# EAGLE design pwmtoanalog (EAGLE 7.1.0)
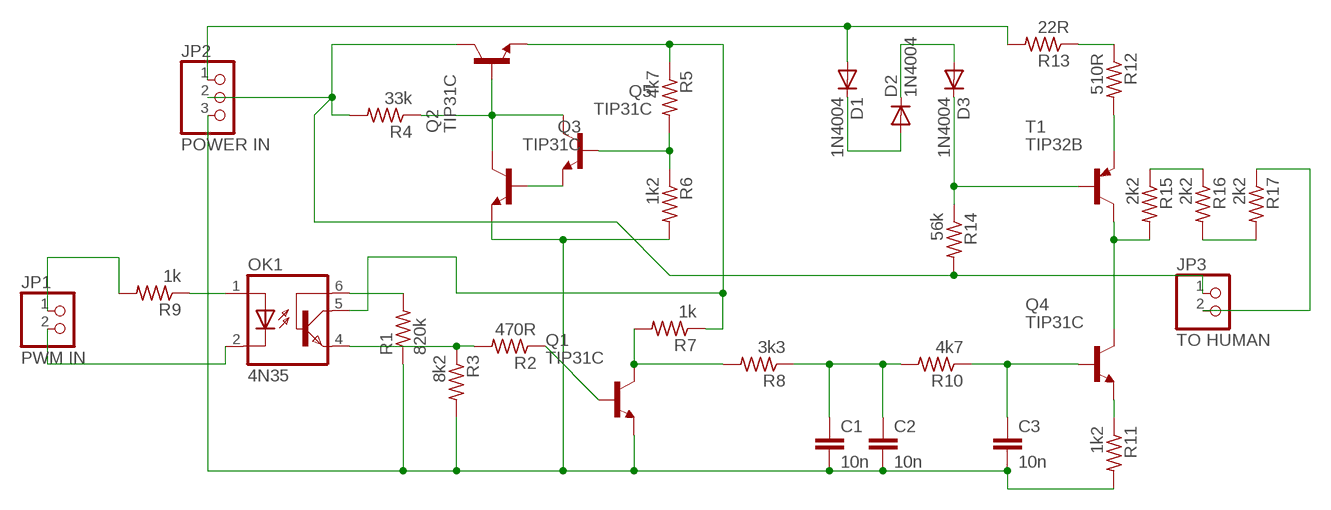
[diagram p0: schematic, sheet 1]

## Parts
C1  10n  C-EU025-030X050  [C025-030X050]
C2  10n  C-EU025-030X050  [C025-030X050]
C3  10n  C-EU025-030X050  [C025-030X050]
D1  1N4004  [DO41-10]
D2  1N4004  [DO41-10]
D3  1N4004  [DO41-10]
JP1  PWM IN  PINHD-1X2  [1X02]
JP2  POWER IN  PINHD-1X3  [1X03]
JP3  TO HUMAN  PINHD-1X2  [1X02]
OK1  4N35  [DIL06]
Q1  TIP31C  [TO220]
Q2  TIP31C  [TO220]
Q3  TIP31C  [TO220]
Q4  TIP31C  [TO220]
Q5  TIP31C  [TO220]
R1  820k  R-US_0207/10  [0207/10]
R2  470R  R-US_0207/10  [0207/10]
R3  8k2  R-US_0207/10  [0207/10]
R4  33k  R-US_0207/10  [0207/10]
R5  4k7  R-US_0207/10  [0207/10]
R6  1k2  R-US_0207/10  [0207/10]
R7  1k  R-US_0207/10  [0207/10]
R8  3k3  R-US_0207/10  [0207/10]
R9  1k  R-US_0207/10  [0207/10]
R10  4k7  R-US_0207/10  [0207/10]
R11  1k2  R-US_0207/10  [0207/10]
R12  510R  R-US_0207/10  [0207/10]
R13  22R  R-US_0207/10  [0207/10]
R14  56k  R-US_0207/10  [0207/10]
R15  2k2  R-US_0207/10  [0207/10]
R16  2k2  R-US_0207/10  [0207/10]
R17  2k2  R-US_0207/10  [0207/10]
T1  TIP32B  [TO220]

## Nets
N$1: OK1.6(BAS) R1.2
N$2: C1.2 C2.2 C3.2 JP2.3 Q1.3(E) Q3.3(E) R1.1 R3.2 R6.2 R11.2
N$3: Q1.1(B) R2.1
N$4: OK1.4(EMI) R2.2 R3.1
N$5: Q2.1(B) Q3.2(C) Q5.2(C) R4.1
N$6: Q3.1(B) Q5.3(E)
N$7: Q5.1(B) R5.2 R6.1
N$8: Q4.3(E) R11.1
N$9: OK1.5(COL) Q2.3(E) R5.1 R7.1
N$10: JP2.2 JP3.1 Q2.2(C) R4.2 R14.2
N$11: Q1.2(C) R7.2 R8.2
N$12: JP1.1 R9.2
N$13: OK1.1(A) R9.1
N$14: JP1.2 OK1.2(C)
N$15: D1.A JP2.1 R13.2
N$16: C3.1 Q4.1(B) R10.1
N$17: C1.1 C2.1 R8.1 R10.2
N$18: R12.1 R13.1
N$19: R12.2 T1.3(E)
N$20: Q4.2(C) R15.2 T1.2(C)
N$21: D3.C R14.1 T1.1(B)
N$22: D1.C D2.A
N$23: D2.C D3.A
N$24: R15.1 R16.1
N$25: R16.2 R17.2
N$26: JP3.2 R17.1

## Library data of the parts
C1-C3 = rcl:C-EU: CAPACITOR, European symbol
D1-D3 = diode:1N4004: DIODE
JP1 JP3 = pinhead:PINHD-1X2: PIN HEADER
JP2 = pinhead:PINHD-1X3: PIN HEADER
OK1 = optocoupler:4N35: MOTOROLA OPTO COUPLER; MF: FAIRCHILD SEMICONDUCTOR; MPN: 4N35; OC_FARNELL: 1328375; OC_NEWARK: 72K9946
Q1-Q5 = transistor-npn:TIP31C*: NPN Transistor
R1-R17 = rcl:R-US_: RESISTOR, American symbol
T1 = transistor:TIP32: PNP Transistor Medium Power Linear Switching Applications Source: http://onsemi.com

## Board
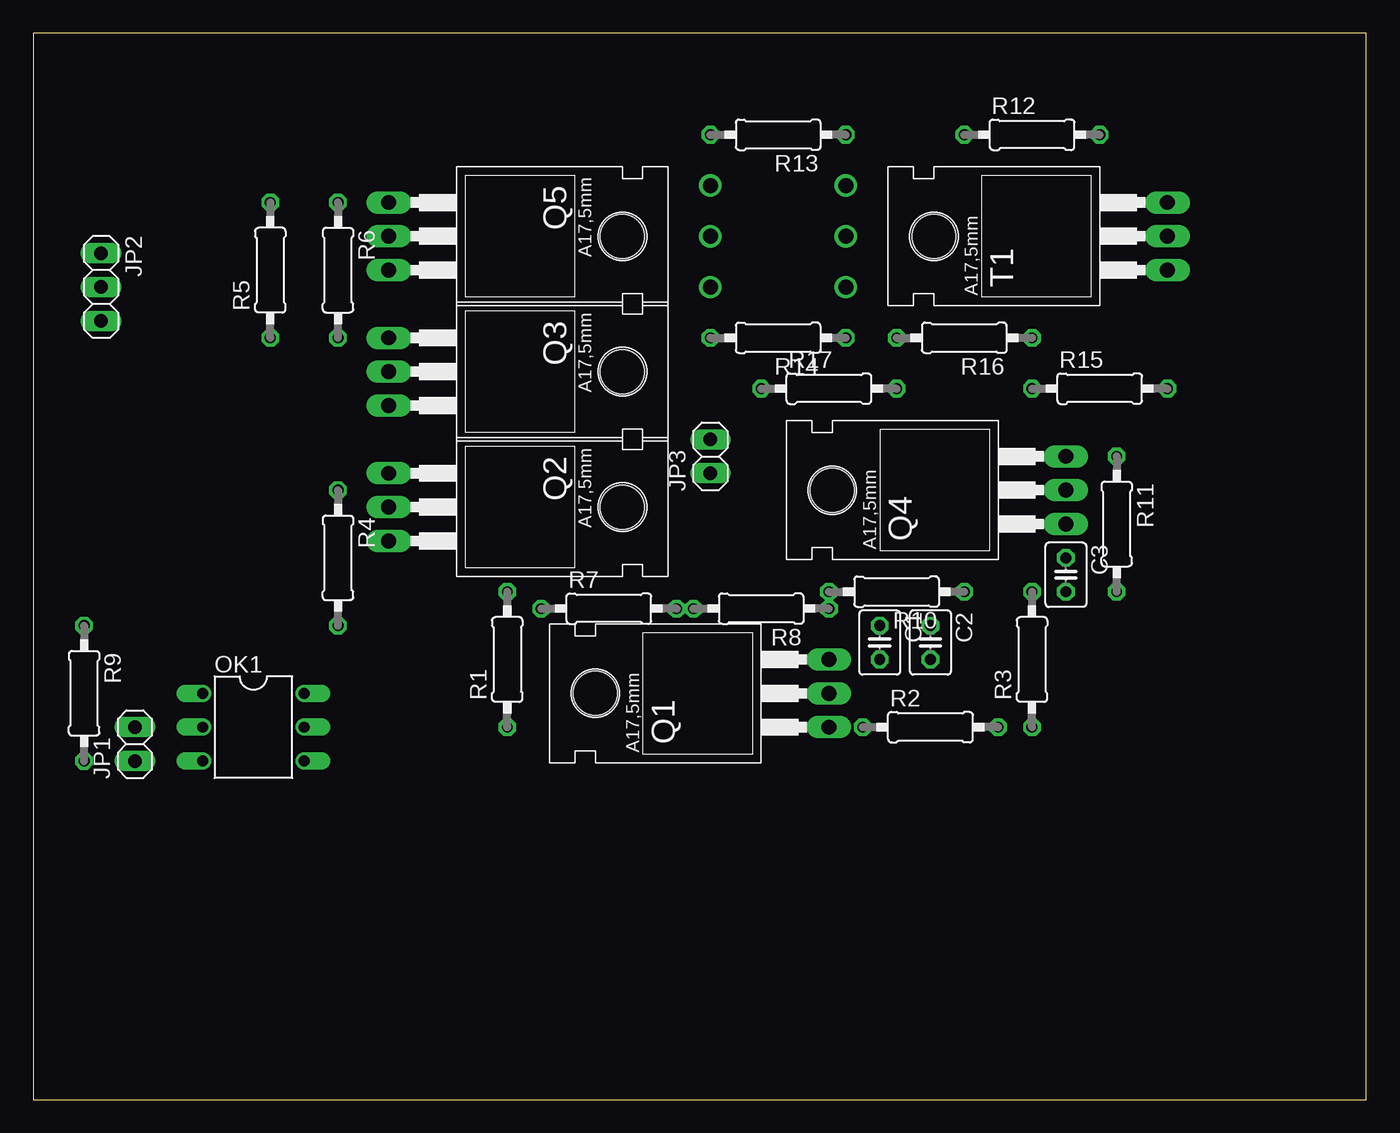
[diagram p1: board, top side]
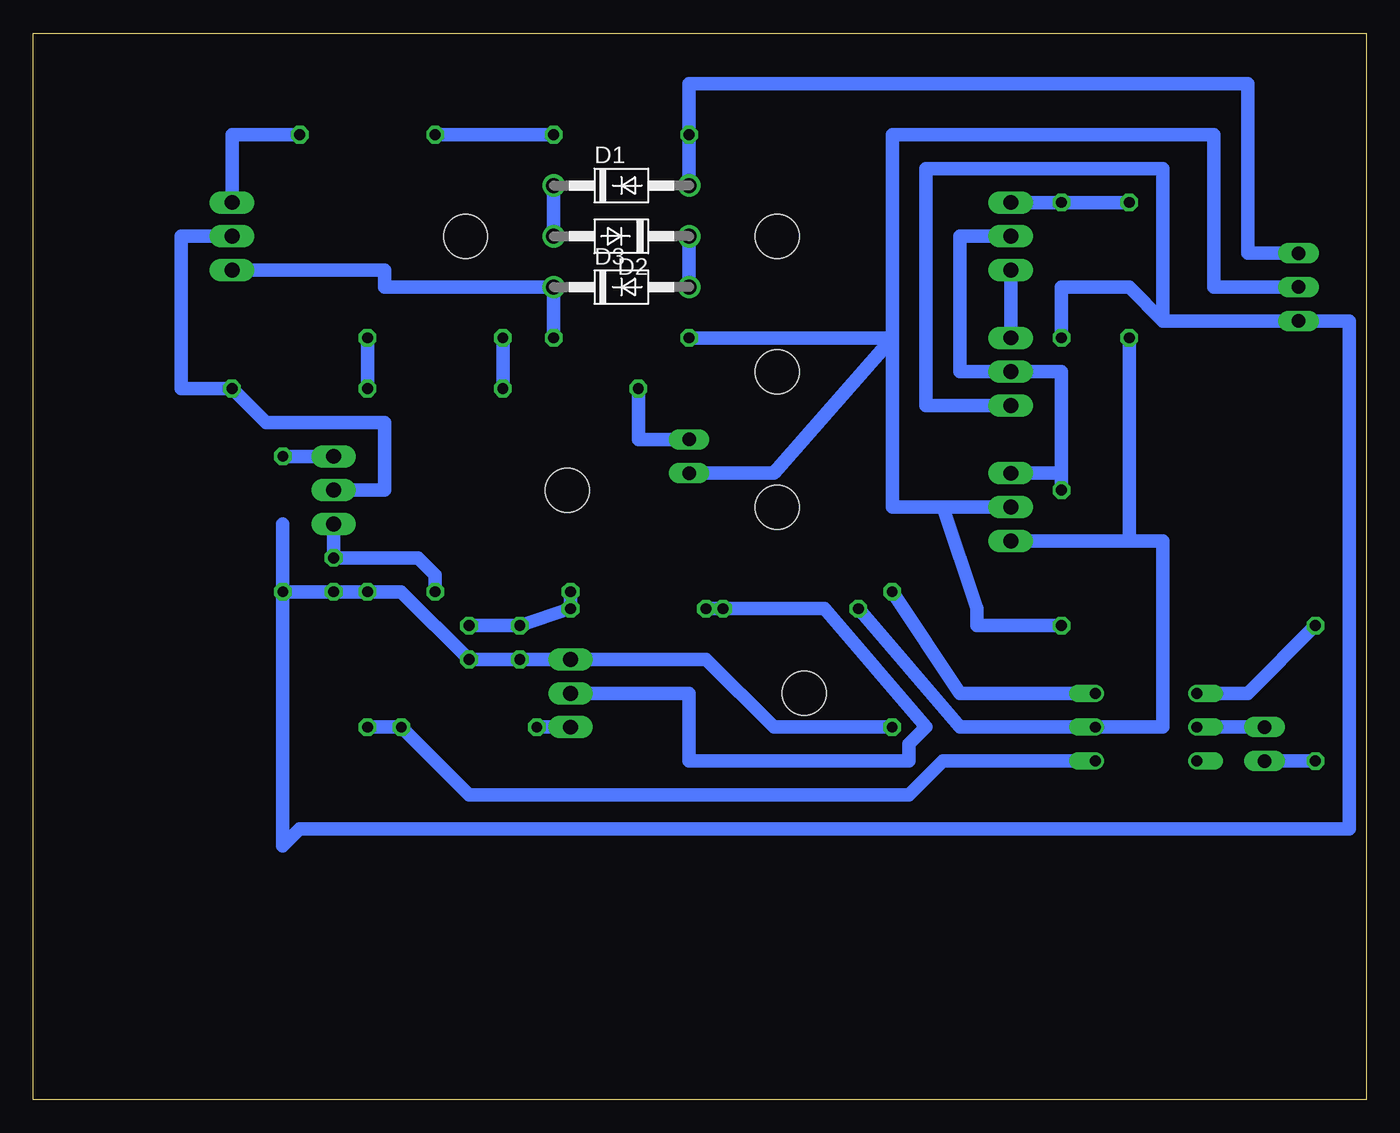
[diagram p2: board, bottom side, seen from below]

Size 100 x 80 mm. Coordinates in mm from the lower left corner, seen from the top.
Outline: 0,0 100,0 100,80 0,80 0,0
Copper layers (1*16): Top 0.035mm / dielectric 1.5mm / Bottom 0.035mm
Design rules "default": minimum track width 10mil, minimum drill 24mil, track to track 8mil, track to pad 8mil, pad to pad 8mil, via to via 8mil, smd to smd 8mil, copper to edge 40mil, drill to drill 8mil, minimum pad ring 10mil, minimum via ring 8mil, stop-mask expansion 4mil, vias tented up to drill 0mil, thermal gap 10mil

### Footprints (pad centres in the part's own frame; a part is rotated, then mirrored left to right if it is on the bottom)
C025-030X050 = drill 0.813 octagon: 1 -1.27,0; 2 1.27,0
DO41-10 = drill 1.118: A 5.08,0; C -5.08,0
1X02 = drill 1.016 long: 1 -1.27,0; 2 1.27,0
1X03 = drill 1.016 long: 1 -2.54,0; 2 0,0; 3 2.54,0
DIL06 = drill 0.813 offset: 1 -2.54,-3.81; 2 0,-3.81; 3 2.54,-3.81; 4 2.54,3.81; 5 0,3.81; 6 -2.54,3.81
TO220 = drill 1.118 long: 1 -2.54,-6.35; 2 0,-6.35; 3 2.54,-6.35 | hole 3.302: 0,11.176
0207/10 = drill 0.813 octagon: 1 -5.08,0; 2 5.08,0

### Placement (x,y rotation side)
C1  63.5,34.29 270 top
C2  67.31,34.29 270 top
C3  77.47,39.37 270 top
D1  55.88,68.58 0 bottom
D2  55.88,64.77 180 bottom
D3  55.88,60.96 0 bottom
JP1  7.62,26.67 90 top
JP2  5.08,60.96 270 top
JP3  50.8,48.26 90 top
OK1  16.51,27.94 270 top
Q1  53.34,30.48 90 top
Q2  33.02,44.45 270 top
Q3  33.02,54.61 270 top
Q4  71.12,45.72 90 top
Q5  33.02,64.77 270 top
R1  35.56,33.02 90 top
R2  67.31,27.94 0 top
R3  74.93,33.02 90 top
R4  22.86,40.64 270 top
R5  17.78,62.23 90 top
R6  22.86,62.23 270 top
R7  43.18,36.83 0 top
R8  54.61,36.83 180 top
R9  3.81,30.48 270 top
R10  64.77,38.1 180 top
R11  81.28,43.18 270 top
R12  74.93,72.39 0 top
R13  55.88,72.39 180 top
R14  55.88,57.15 180 top
R15  80.01,53.34 0 top
R16  69.85,57.15 180 top
R17  59.69,53.34 0 top
T1  78.74,64.77 90 top

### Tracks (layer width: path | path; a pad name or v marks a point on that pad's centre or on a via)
N$1
  Bottom 1: R1.2 30.48,30.48 OK1.6
N$2
  Bottom 1: R1.1 44.45,27.94 49.53,33.02 Q1.3 C1.2 C2.2 72.39,38.1 R3.2 C3.2 R11.2 | 81.28,43.18 R11.2 | R11.2 81.28,19.05 80.01,20.32 1.27,20.32 1.27,58.42 JP2.3 15.24,58.42 | 15.24,58.42 17.78,60.96 22.86,60.96 R6.2 | Q3.3 33.02,52.07 33.02,69.85 15.24,69.85 15.24,58.42
N$3
  Bottom 1: R2.1 Q1.1
N$4
  Bottom 1: OK1.4 31.75,25.4 34.29,22.86 67.31,22.86 R2.2 R3.1
N$5
  Bottom 1: Q2.1 22.86,46.99 R4.1 22.86,54.61 Q3.2 30.48,54.61 30.48,64.77 Q5.2
N$6
  Bottom 1: Q5.3 Q3.1
N$7
  Bottom 1: R5.2 R6.1 Q5.1
N$8
  Bottom 1: R11.1 Q4.3
N$9
  Bottom 1: R5.1 17.78,41.91 | 17.78,41.91 Q2.3 | R7.1 30.48,27.94 OK1.5 | OK1.5 19.05,27.94 | 17.78,41.91 15.24,41.91 15.24,27.94 OK1.5
N$10
  Bottom 1: 31.75,44.45 29.21,36.83 29.21,35.56 R4.2 | 31.75,44.45 Q2.2 | JP2.2 11.43,60.96 11.43,72.39 35.56,72.39 35.56,57.15 | 35.56,57.15 35.56,44.45 31.75,44.45 | R14.2 35.56,57.15 | JP3.1 44.45,46.99 35.56,57.15
N$11
  Bottom 1: Q1.2 50.8,30.48 50.8,25.4 34.29,25.4 34.29,26.67 33.02,27.94 40.64,36.83 R7.2 R8.2
N$12
  Bottom 1: JP1.1 R9.2
N$13
  Bottom 1: R9.1 8.89,30.48 OK1.1
N$14
  Bottom 1: OK1.2 JP1.2
N$15
  Bottom 1: JP2.1 8.89,63.5 8.89,76.2 50.8,76.2 R13.2 D1.A
N$16
  Bottom 1: R10.1 69.85,39.37 71.12,40.64 C3.1 Q4.1
N$17
  Bottom 1: C2.1 C1.1 R8.1 R10.2
N$18
  Bottom 1: R13.1 R12.1
N$19
  Bottom 1: R12.2 85.09,72.39 T1.3
N$20
  Bottom 1: T1.2 88.9,64.77 88.9,53.34 R15.2 82.55,50.8 73.66,50.8 73.66,45.72 Q4.2
N$21
  Bottom 1: T1.1 73.66,62.23 73.66,60.96 D3.C R14.1
N$22
  Bottom 1: D1.C D2.A
N$23
  Bottom 1: D2.C D3.A
N$24
  Bottom 1: R16.1 R15.1
N$25
  Bottom 1: R16.2 R17.2
N$26
  Bottom 1: R17.1 54.61,49.53 JP3.2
